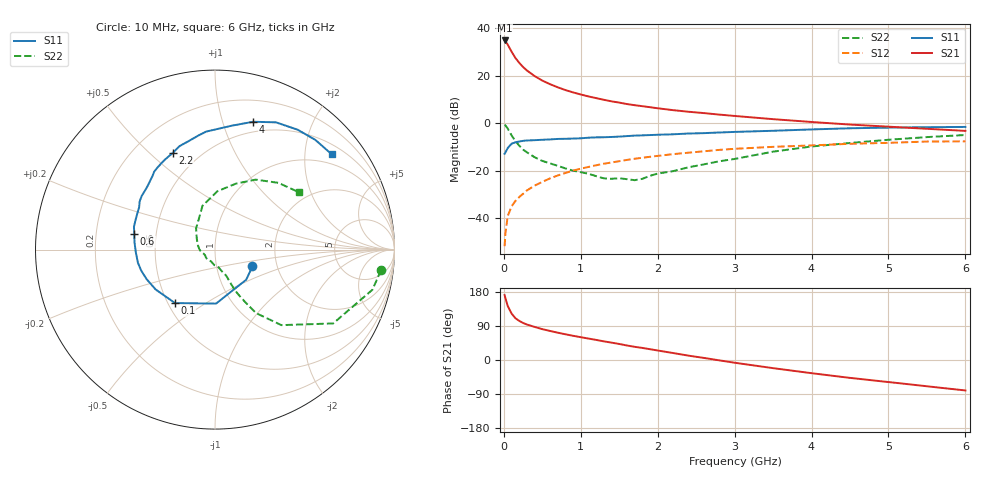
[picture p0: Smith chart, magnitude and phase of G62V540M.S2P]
! SIEMENS Small Signal Semiconductors
! BFG193
! Si NPN RF Bipolar Junction Transistor in SOT223
! VCE = 2.5 V  IC = 40 mA
! Common Emitter S-Parameters:  August  1996
# GHz  S  MA  R  50
!  f  S11  S21  S12  S22
! GHz  MAG  ANG  MAG  ANG  MAG  ANG  MAG  ANG
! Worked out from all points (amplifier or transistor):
!   36 points, 10 MHz to 6 GHz, reference 50 ohm
!   highest |S21| = 34.9 dB at 10 MHz (marker M1)
!   |S21| within 3 dB of that: start of sweep to 71.56 MHz
!   unconditionally stable (mu >= 1): 463.2 MHz to 2.449 GHz
!   at 250 MHz: K = 0.90, MSG = 26.7 dB, |S12| = -29.7 dB
!   at 1.4 GHz: K = 1.05, MAG = 11.5 dB, |S12| = -16.5 dB
!   at 6 GHz: K = 0.91, MSG = 2.2 dB, |S12| = -7.6 dB
!   S11 on the Smith chart (normalised r, x): 10 MHz: 1.49, -0.29; 100 MHz: 0.54, -0.38; 600 MHz: 0.37, +0.08; 2.2 GHz: 0.36, +0.59; 4 GHz: 0.40, +1.26; 6 GHz: 0.73, +2.63
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0.01  0.2288 -24.1  55.39 171.3  0.0026 87.7  0.932 -7.1
0.02  0.2416 -44.0  53.67 163.5  0.0047 80.5  0.9052 -14.3
0.05  0.3009 -88.9  45.41 142.7  0.0111 70.4  0.7763 -32.0
0.1  0.372 -126.8  32.31 122.8  0.0178 65.5  0.5602 -48.7
0.15  0.3984 -146.1  23.78 110.3  0.0232 64.1  0.4215 -57.1
0.2  0.415 -156.6  18.74 103.2  0.0281 65.0  0.3402 -60.0
0.25  0.4276 -164.2  15.3 97.7  0.0328 66.1  0.2803 -62.6
0.3  0.4357 -170.3  12.94 93.6  0.0387 67.0  0.2455 -64.1
0.4  0.4417 -178.3  9.865 87.3  0.0488 67.4  0.1935 -65.5
0.5  0.4506 174.6  7.926 81.4  0.0586 66.9  0.1618 -66.5
0.6  0.4583 169.0  6.663 76.7  0.0693 65.9  0.1435 -68.6
0.8  0.4724 159.7  5.01 67.9  0.0901 62.7  0.1125 -75.6
1.1  0.498 147.5  3.68 56.6  0.1208 57.6  0.0869 -92.2
1.3  0.5093 140.5  3.124 49.2  0.1411 53.5  0.0695 -107.9
1.6  0.5383 130.3  2.542 38.3  0.1698 46.6  0.0668 -139.2
2.2  0.5875 113.7  1.892 18.4  0.2246 32.9  0.0985 165.5
2.8  0.6411 98.6  1.526 -0.9  0.2759 18.8  0.1589 131.6
3.5  0.6966 82.3  1.223 -21.5  0.3198 1.5  0.2534 106.0
4  0.7433 73.4  1.067 -34.8  0.3424 -8.4  0.3254 87.7
4.5  0.7862 64.4  0.941 -47.2  0.371 -18.5  0.3856 72.4
5.5  0.8284 47.5  0.767 -69.3  0.4134 -41.6  0.5128 46.5
6  0.8396 39.2  0.693 -80.4  0.4176 -54.8  0.5679 34.1
